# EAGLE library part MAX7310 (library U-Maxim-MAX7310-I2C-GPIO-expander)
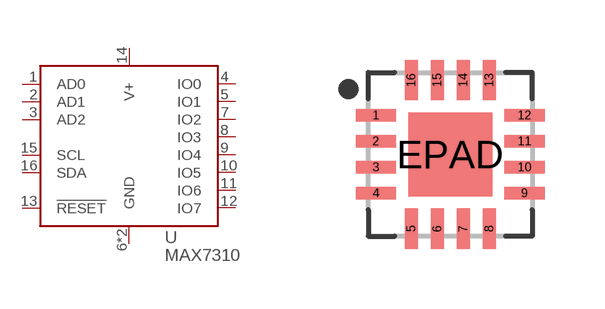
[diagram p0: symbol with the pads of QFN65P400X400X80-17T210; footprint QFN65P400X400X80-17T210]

Designator prefix U

## MAX7310  [QFN65P400X400X80-17T210]
1  AD0  in
2  AD1  in
3  AD2  in
4  IO0
5  IO1
6  GND  pwr
7  IO2
8  IO3
9  IO4
10  IO5
11  IO6
12  IO7
13  !RESET  in
14  V+  pwr
15  SCL  in
16  SDA
EPAD  GND  pwr

## Footprint QFN65P400X400X80-17T210 (pad centres in mm)
16-QFN, 0.65 mm pitch, 4.00 X 4.00 X 0.80 mm body, 2.10 X 2.10 mm thermal pad 16-pin QFN package with 0.65 mm pitch with body size 4.00 X 4.00 X 0.80 mm and thermal pad size 2.10 X 2.10 mm
smd 1.01 x 0.32: 1 -1.86,0.975; 2 -1.86,0.325; 3 -1.86,-0.325; 4 -1.86,-0.975; 9 1.86,-0.975; 10 1.86,-0.325; 11 1.86,0.325; 12 1.86,0.975
smd 0.32 x 1.01: 5 -0.975,-1.86; 6 -0.325,-1.86; 7 0.325,-1.86; 8 0.975,-1.86; 13 0.975,1.86; 14 0.325,1.86; 15 -0.325,1.86; 16 -0.975,1.86
smd 2.1 x 2.1: EPAD 0,0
